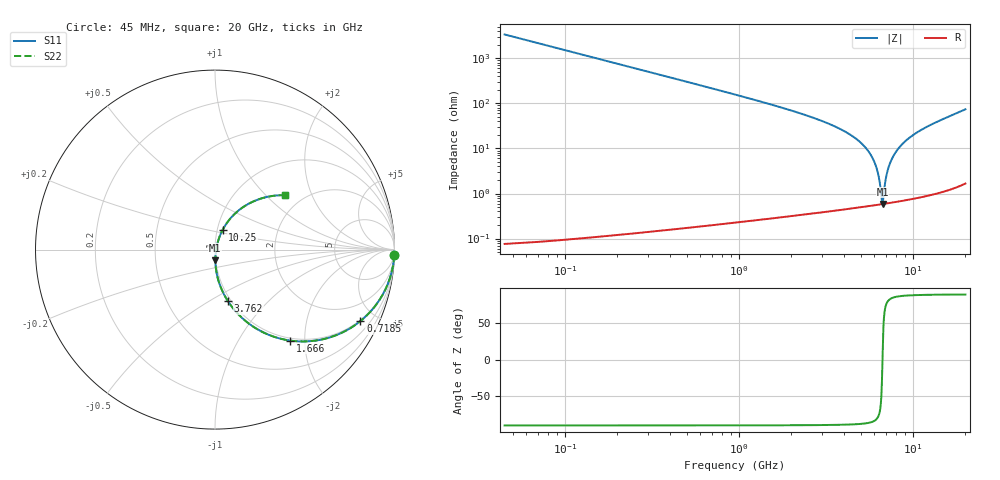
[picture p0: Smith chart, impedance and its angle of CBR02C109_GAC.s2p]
! S-parameter model data by Modelithics Inc.  support@modelithics.com 813-866-6335  Tampa FL USA
! S-Parameter data specifications:
! Substrate: 20-mil Rogers 4350B, substrate thickness, H=0.508mm, Dielectric constant, Er=3.75
! PCB Mounting Pad Footprint: Pad width, PadW=0.32mm , Pad length, PadL=0.37mm , Pad gap, PadG (edge-to-edge)=0.19mm , Reference planes=0.93mm apart
#  GHz  S  MA  R 50
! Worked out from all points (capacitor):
!   801 points, 45 MHz to 20 GHz, reference 50 ohm
!   read as one part in series: C = 1.04 pF near 144.8 MHz
!   lowest |Z| = 584 mohm at 6.68 GHz (marker M1)
!   series resonance near 6.677 GHz, so ESL is about 540 pH
!   S11 on the Smith chart (normalised r, x): 45 MHz: 1, -66; 718.5 MHz: 0.95, -4.09; 1.666 GHz: 0.95, -1.70; 3.762 GHz: 0.97, -0.61; 10.25 GHz: 1.06, +0.24; 20 GHz: 1.63, +1.31
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0.045  0.9996 -1.7  0.02953 88.3  0.02953 88.3  0.9996 -1.7
0.194662  0.9919 -7.5  0.1268 82.5  0.1268 82.5  0.9919 -7.5
0.294438  0.9817 -11.3  0.19 78.7  0.19 78.7  0.9817 -11.3
0.469044  0.9553 -17.7  0.2952 72.3  0.2952 72.3  0.9553 -17.7
0.718481  0.9027 -26.2  0.4293 63.8  0.4293 63.8  0.9027 -26.2
1.666344  0.6568 -50.5  0.7519 39.3  0.7519 39.3  0.6568 -50.5
2.4396  0.4906 -62.8  0.8684 26.8  0.8684 26.8  0.4906 -62.8
3.387462  0.3431 -72.8  0.9355 16.5  0.9355 16.5  0.3431 -72.8
3.761619  0.2973 -75.9  0.9507 13.4  0.9507 13.4  0.2973 -75.9
5.582512  0.1325 -86.0  0.9859 1.8  0.9859 1.8  0.1325 -86.0
6.680038  0.06041 -88.1  0.9923 -3.5  0.9923 -3.5  0.06041 -88.1
6.704981  0.05892 -88.0  0.9924 -3.6  0.9924 -3.6  0.05892 -88.0
7.253744  0.02765 -83.4  0.9935 -6.0  0.9935 -6.0  0.02765 -83.4
7.752619  0.006306 -8.4  0.9936 -8.1  0.9936 -8.1  0.006306 -8.4
8.176663  0.02269 63.5  0.9931 -9.8  0.9931 -9.8  0.02269 63.5
8.550819  0.04077 69.3  0.9923 -11.2  0.9923 -11.2  0.04077 69.3
9.149469  0.06893 70.7  0.9904 -13.5  0.9904 -13.5  0.06893 70.7
10.0225  0.1081 69.4  0.9865 -16.6  0.9865 -16.6  0.1081 69.4
10.24699  0.1178 68.9  0.9853 -17.4  0.9853 -17.4  0.1178 68.9
13.36496  0.2445 59.7  0.9601 -28.1  0.9601 -28.1  0.2445 59.7
16.68248  0.371 49.0  0.9168 -39.2  0.9168 -39.2  0.371 49.0
20  0.4957 37.7  0.8536 -50.6  0.8536 -50.6  0.4957 37.7
